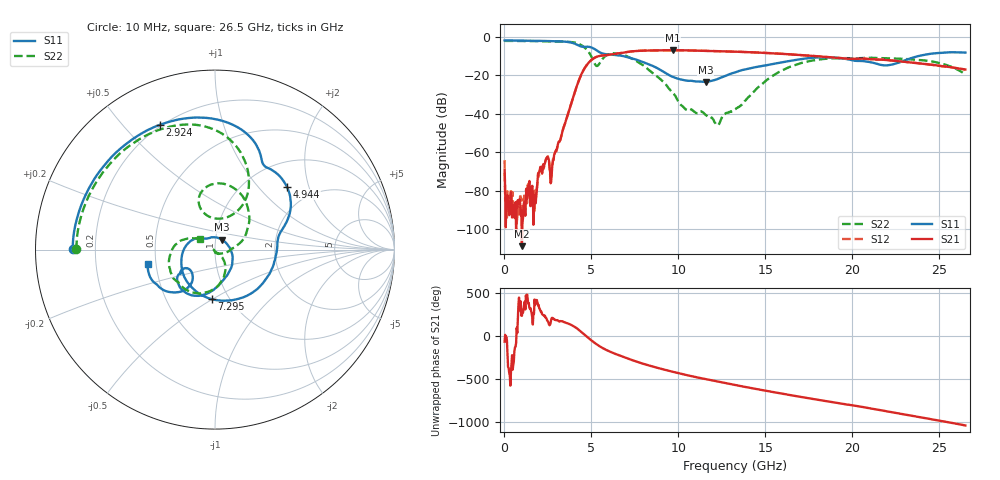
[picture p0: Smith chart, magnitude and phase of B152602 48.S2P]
!  2-Port S-parameters saved by WinCal
! VAR MeasName=S-Parameters (CALIBRATED_DATA) read from VNA (N5242A)
! VAR MeasDate=2016-1-5 16:32:59
! VAR NAME=B152602 48
! VAR FILENAME=B152602 48.S2P
! VAR DATE=2016-1-5 16:32:59
! VAR PHYS_PORTS=1,2
# Hz S DB R 50
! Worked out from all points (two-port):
!   801 points, 10 MHz to 26.5 GHz, reference 50 ohm
!   highest |S21| = -7.08 dB at 9.679 GHz (marker M1); lowest = -108.7 dB at 1.003 GHz (marker M2)
!   |S21| within 3 dB of the highest: 5.451 GHz to 17.77 GHz (12.31 GHz wide, 106 % of centre)
!   lowest |S11| = -23.5 dB at 11.57 GHz (marker M3), VSWR 1.14, Z = 53.4 + j5.99 ohm
!   |S11| at or under -10 dB: 6.765 GHz to 23.85 GHz (17.09 GHz wide, 112 % of centre)
!   |S22| runs from -45.9 to -2.2 dB; largest |S21 - S12| = 0.0032
!   S11 on the Smith chart (normalised r, x): 10 MHz: 0.12, +0.00; 2.924 GHz: 0.19, +0.63; 4.944 GHz: 1.48, +1.45; 7.295 GHz: 0.83, -0.50; 26.5 GHz: 0.45, -0.08
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1e7  -2.02 179.8  -69.26 -66.0  -64.09 -4.5  -2.24 179.8
1.755625e8  -2.02 176.3  -82.20 152.9  -80.25 159.0  -2.24 177.3
1.003375e9  -2.12 159.4  -108.71 -124.4  -89.07 15.7  -2.29 164.5
1.764962e9  -2.21 143.2  -84.11 7.6  -79.78 -11.3  -2.37 152.2
2.096088e9  -2.24 135.6  -67.59 -77.4  -68.78 -79.7  -2.40 146.5
2.427212e9  -2.29 127.6  -62.78 -159.8  -63.30 -156.0  -2.44 140.5
2.725225e9  -2.33 119.7  -69.87 -148.9  -68.46 -150.4  -2.46 134.7
2.9239e9  -2.38 114.0  -59.95 -172.5  -59.66 -172.0  -2.50 130.5
4.447075e9  -5.22 60.9  -19.12 42.3  -19.12 42.4  -4.59 78.6
4.943762e9  -5.47 41.3  -12.59 -42.7  -12.60 -42.6  -9.44 58.9
5.341112e9  -7.43 20.8  -10.35 -102.9  -10.35 -102.8  -15.20 90.4
6.036475e9  -9.29 -3.0  -9.46 179.6  -9.46 179.7  -9.04 97.5
7.29475e9  -11.16 -93.9  -7.68 81.2  -7.68 81.2  -11.23 46.3
8.851038e9  -16.68 162.3  -7.16 -15.3  -7.15 -15.5  -21.21 -0.6
9.67885e9  -20.85 136.4  -7.08 -58.5  -7.09 -58.5  -29.25 -41.4
1.156626e10  -23.53 56.9  -7.39 -144.7  -7.40 -144.7  -40.57 -176.1
1.226162e10  -21.94 12.2  -7.54 -173.4  -7.54 -173.3  -45.79 -130.8
1.3255e10  -18.60 -34.4  -7.83 147.3  -7.83 147.4  -37.78 -83.4
1.504308e10  -14.90 -76.7  -8.49 79.8  -8.48 79.6  -22.81 -50.2
1.769208e10  -11.00 -114.3  -10.01 -14.6  -9.98 -14.5  -12.45 -99.4
2.209604e10  -14.81 -135.3  -12.28 -164.3  -12.23 -164.6  -11.28 -157.8
2.65e10  -8.30 -168.0  -17.08 34.6  -17.09 34.4  -19.75 146.6
